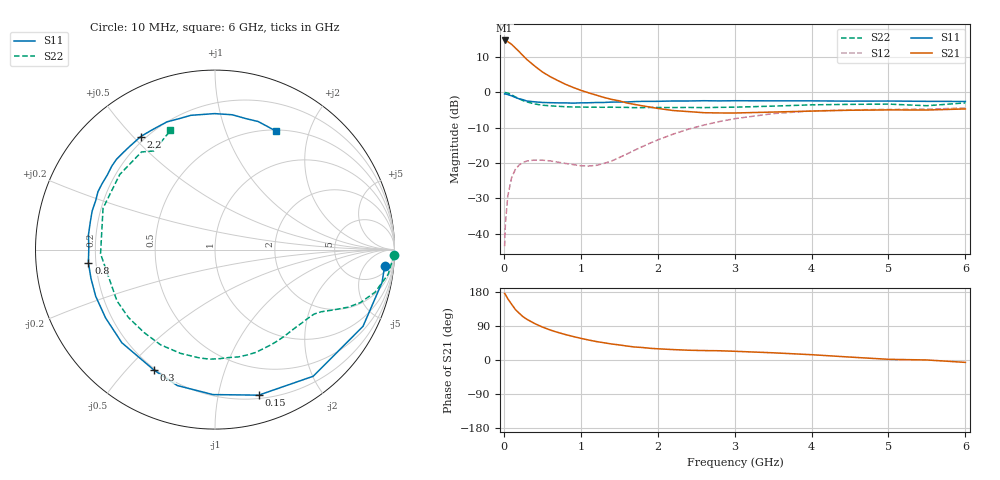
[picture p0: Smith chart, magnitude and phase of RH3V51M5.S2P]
! SIEMENS Small Signal Semiconductors
! BFR106
! Si NPN RF Bipolar Junction Transistor in SOT23
! VCE = 3.5 V  IC = 1.5 mA
! Common Emitter S-Parameters:  August  1996
# GHz  S  MA  R  50
!  f  S11  S21  S12  S22
! GHz  MAG  ANG  MAG  ANG  MAG  ANG  MAG  ANG
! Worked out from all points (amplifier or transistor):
!   36 points, 10 MHz to 6 GHz, reference 50 ohm
!   highest |S21| = 14.7 dB at 10 MHz (marker M1)
!   |S21| within 3 dB of that: start of sweep to 191.9 MHz
!   unconditionally stable (mu >= 1): 820.2 MHz to 2.006 GHz; 3.293 GHz to end of sweep
!   at 250 MHz: K = 0.28, MSG = 15.1 dB, |S12| = -19.8 dB
!   at 1.4 GHz: K = 1.33, MAG = 5.3 dB, |S12| = -19.4 dB
!   at 6 GHz: K = 1.02, MAG = -1.0 dB, |S12| = -4.4 dB
!   S11 on the Smith chart (normalised r, x): 10 MHz: 9, -16; 150 MHz: 0.23, -1.32; 300 MHz: 0.19, -0.60; 800 MHz: 0.17, -0.05; 2.2 GHz: 0.18, +0.53; 6 GHz: 0.51, +1.51
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0.01  0.9496 -5.5  5.403 175.8  0.0067 86.6  0.9997 -1.8
0.02  0.9487 -11.1  5.373 173.1  0.0135 86.3  0.9911 -3.3
0.05  0.9288 -27.4  5.204 162.1  0.0336 74.7  0.9746 -8.1
0.1  0.893 -52.2  4.77 147.4  0.0616 62.0  0.9227 -14.9
0.15  0.8466 -73.3  4.235 133.2  0.0814 50.6  0.8625 -20.0
0.2  0.8078 -90.8  3.75 123.3  0.0941 43.1  0.8097 -23.3
0.25  0.7861 -105.5  3.288 114.1  0.102 36.4  0.7637 -25.7
0.3  0.7526 -116.8  2.904 107.3  0.1069 32.1  0.7315 -27.5
0.4  0.734 -135.0  2.356 96.3  0.1105 25.7  0.6848 -30.4
0.5  0.7187 -148.0  1.942 87.0  0.1099 22.2  0.6581 -33.1
0.6  0.7138 -158.6  1.67 79.4  0.1074 20.6  0.6445 -36.3
0.8  0.7091 -174.1  1.301 67.2  0.0989 22.8  0.6258 -43.3
1.1  0.7116 167.5  0.985 52.8  0.0908 37.6  0.6166 -55.2
1.6  0.7301 145.2  0.706 36.8  0.1345 66.8  0.6121 -77.7
2.2  0.7539 123.3  0.553 27.5  0.2564 68.3  0.6091 -108.3
2.8  0.7564 105.2  0.511 24.4  0.3855 55.5  0.613 -141.9
3.5  0.7577 90.2  0.526 19.0  0.5003 37.9  0.638 -177.9
4  0.7573 82.7  0.543 14.0  0.5451 26.1  0.6651 159.7
4.5  0.7499 76.6  0.558 7.7  0.5645 16.0  0.6758 141.7
5  0.753 71.4  0.564 1.8  0.5731 7.8  0.681 127.0
5.5  0.7452 66.6  0.562 0.1  0.5774 3.9  0.6466 121.8
6  0.7425 63.0  0.582 -6.3  0.6006 -4.0  0.7088 110.5
